PROGRAM MAIN
VAR
	axis1: Axis_PTP_CoE;	
    home_exe AT%I*:BOOL;
    mstep:manualstep;
	AutoMode: BOOL;
END_VAR

axis1.sName:="X轴";
axis1.areset( );                                //刷新IO，读取轴状态、复位
axis1.aPower( );                                //使能

IF axis1.Ref.Status.ControlLoopClosed AND NOT AutoMode THEN      //判断使能成功，调用手动模式下点动指令
axis1.aManualJOG(Velo:=100 ,);
END_IF


IF home_exe THEN axis1.aHome(execute:=TRUE);  
	ELSE axis1.aHome(execute:=FALSE);
END_IF

IF automode THEN                              //自动模式下的指令使用
logic();
END_IF

ACTION logic:
CASE mstep OF 
	moveoff:
	   axis1.aStop(execute:=FALSE);
	   axis1.aMoveOff();
	jogB:
	   axis1.aJogB(execute:=TRUE,velo:=100); 
	jogF:
	   axis1.aJogF(execute:=TRUE,velo:=100); 
    homing:  
       axis1.aHome(execute:=TRUE);
       IF axis1.done THEN
	    mstep:=moveoff;
       END_IF
	MoveRel:
	   axis1.aMoverel(execute:=TRUE,Target:=100,velo:=100);
	   IF axis1.done THEN
	    mstep:=moveoff;
	   END_IF
	Moveabs:
	   axis1.aMoveabs(execute:=TRUE,Target:=100,velo:=100);
	   IF axis1.done THEN
	    mstep:=moveoff;
	   END_IF
	MoveVel:
	   axis1.aMoveVel(execute:=TRUE,velo:=100);
    stop:
	   axis1.aStop(execute:=TRUE);
END_CASE
END_ACTION

END_PROGRAM
